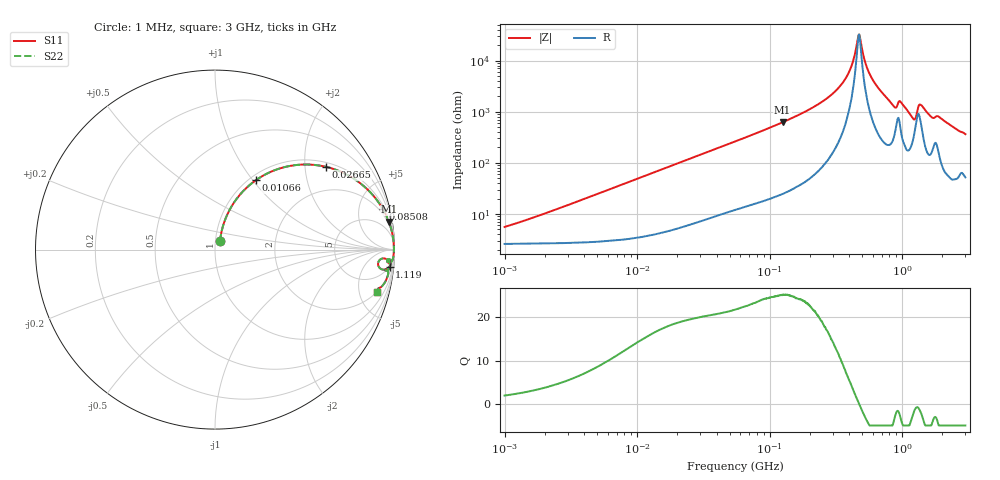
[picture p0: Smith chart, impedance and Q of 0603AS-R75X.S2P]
!s-Parameter Generated by FASTRON Sdn. Bhd.
!FASTRON P/N : 0603AS-R75X
!Keysight Technologies: E4991B_MY54100416_A.01.15
!Date created: Tue Oct 17 15:45:28 2023
!Version  : Rev01 Tue Oct 17 15:45:28 2023
!Data & Calibration Information:
!Freq	S11	S21	S12	S22
!PortZ  Port1:50+j0  Port2:50+j0
!When reading reference impedance value at option line is always used.
! Remarks : This data is being provided solely for informational purposes.
# Hz S dB R 50
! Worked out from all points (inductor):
!   1601 points, 1 MHz to 3 GHz, reference 50 ohm
!   read as one part in series: L = 783 nH near 1.609 MHz
!   highest Q = 25.2 at 125.1 MHz (marker M1), where L = 789 nH
!   self-resonance near 471 MHz
!   S11 on the Smith chart (normalised r, x): 1 MHz: 1.05, +0.10; 10.66 MHz: 1.07, +1.04; 26.65 MHz: 1.13, +2.57; 85.08 MHz: 1.34, +8.18; 1.119 GHz: 5, -19; 3 GHz: 2.04, -7.22
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1000000  -25.27 59.5  -0.23 -2.8  -0.23 -2.8  -25.27 59.5
3804036  -14.87 71.2  -0.38 -10.3  -0.38 -10.3  -14.87 71.2
1.066409e7  -6.95 59.5  -1.28 -26.6  -1.28 -26.6  -6.95 59.5
1.447069e7  -5.03 52.6  -1.98 -34.0  -1.98 -34.0  -5.03 52.6
2.664524e7  -2.27 36.8  -4.44 -50.3  -4.44 -50.3  -2.27 36.8
5.477226e7  -0.72 20.6  -9.07 -66.8  -9.07 -66.8  -0.72 20.6
8.507507e7  -0.33 13.6  -12.58 -74.0  -12.58 -74.0  -0.33 13.6
1.250659e8  -0.16 9.1  -16.02 -78.6  -16.02 -78.6  -0.16 9.1
2.083556e8  -0.06 4.8  -21.51 -82.6  -21.51 -82.6  -0.06 4.8
3.631036e8  -0.03 1.4  -31.98 -81.8  -31.98 -81.8  -0.03 1.4
4.135554e8  -0.03 0.7  -37.72 -76.1  -37.72 -76.1  -0.03 0.7
4.710174e8  -0.03 0.0  -50.17 -6.2  -50.17 -6.2  -0.03 0.0
5.753936e8  -0.03 -1.1  -34.19 78.4  -34.19 78.4  -0.03 -1.1
7.925923e8  -0.08 -3.3  -24.60 79.0  -24.60 79.0  -0.08 -3.3
8.804142e8  -0.24 -4.3  -21.96 67.5  -21.96 67.5  -0.24 -4.3
9.730857e8  -0.18 -3.4  -24.07 69.6  -24.07 69.6  -0.18 -3.4
1.11944e9  -0.20 -5.6  -20.01 74.0  -20.01 74.0  -0.20 -5.6
1.231095e9  -0.66 -6.5  -17.62 53.2  -17.62 53.2  -0.66 -6.5
1.381259e9  -0.30 -3.6  -22.99 59.5  -22.99 59.5  -0.30 -3.6
1.662201e9  -0.28 -6.9  -18.22 71.7  -18.22 71.7  -0.28 -6.9
1.883708e9  -0.27 -6.8  -18.35 71.9  -18.35 71.9  -0.27 -6.8
3e9  -0.62 -14.6  -11.85 67.2  -11.85 67.2  -0.62 -14.6
